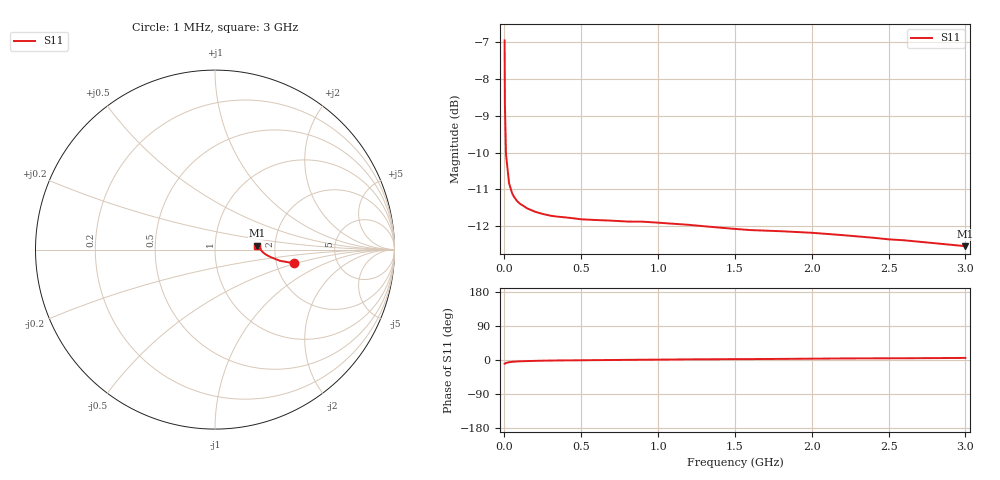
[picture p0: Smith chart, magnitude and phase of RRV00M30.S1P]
! SIEMENS Small Signal Semiconductors
! BA595
! Si PIN Diode in SOD323
! IF = 0.3 mA
! S-Parameters:  July  1992
# GHz  S  MA  R  50
!  f  S11
! GHz  MAG  ANG
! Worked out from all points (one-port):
!   33 points, 1 MHz to 3 GHz, reference 50 ohm
!   lowest |S11| = -12.5 dB at 3 GHz (marker M1), VSWR 1.62, Z = 80.6 + j3.86 ohm
!   |S11| at or under -10 dB: 9.782 MHz to end of sweep
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0.001  0.4492 -9.8
0.003  0.3677 -9.8
0.01  0.3147 -7.8
0.03  0.2873 -5.8
0.05  0.2784 -4.8
0.06  0.2758 -4.5
0.08  0.272 -3.9
0.1  0.2695 -3.5
0.15  0.2654 -2.8
0.2  0.2627 -2.3
0.25  0.2609 -1.8
0.3  0.2595 -1.5
0.35  0.2587 -1.2
0.4  0.2581 -1.0
0.5  0.2566 -0.7
0.8  0.2548 0.4
0.9  0.2547 0.7
1.2  0.2522 1.7
1.5  0.249 2.3
1.6  0.2481 2.4
1.8  0.2472 2.9
2  0.246 3.5
2.2  0.2442 4.1
2.4  0.2422 4.4
2.5  0.241 4.5
2.6  0.2403 4.6
2.8  0.2381 5.0
3  0.2359 5.5
